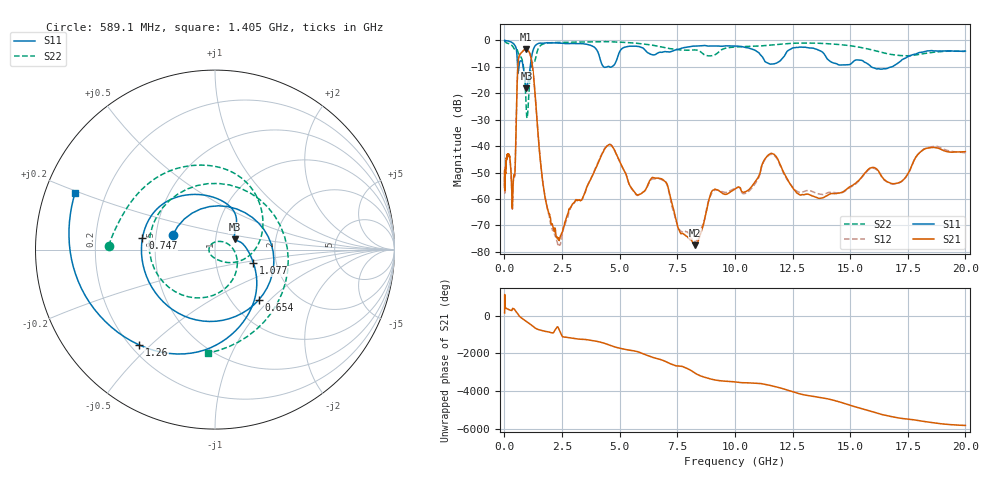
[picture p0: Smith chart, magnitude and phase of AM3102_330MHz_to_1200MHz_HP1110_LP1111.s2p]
! Date/Time: Tue, Sep 11, 2018 5:23 PM
! Network Analyzer: Agilent Technologies E8362B Rev: A.07.50.63
! Sweep from 0.010 to 20.000 GHz, 1601 Points, Sweep Type: LOG
! Power Supply: 4.949 V, 0.001 A
# Hz S DB R 50
!freq MagS11 AngS11 MagS21 AngS21 MagS12 AngS12 MagS22 AngS22
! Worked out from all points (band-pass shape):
!   1601 points, 10 MHz to 20 GHz, reference 50 ohm
!   highest |S21| = -3.32 dB at 920.7 MHz (marker M1); lowest = -77.5 dB at 8.266 GHz (marker M2)
!   |S21| within 3 dB of the highest: 627.8 MHz to 1.15 GHz (521.9 MHz wide, 58.7 % of centre)
!   lowest |S11| = -18.1 dB at 956.4 MHz (marker M3), VSWR 1.29, Z = 61.9 + j7.36 ohm
!   |S11| at or under -10 dB: 815.9 MHz to 1.118 GHz (302.1 MHz wide, 31.2 % of centre); 4.303 GHz to 4.466 GHz (163.1 MHz wide, 3.72 % of centre); 15.92 GHz to 16.81 GHz (892.5 MHz wide, 5.45 % of centre)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
!   |S22| runs from -29.5 to -0.2 dB; largest |S21 - S12| = 0.0084
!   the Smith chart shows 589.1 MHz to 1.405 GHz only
!   S11 on the Smith chart (normalised r, x): 589.1 MHz: 0.61, +0.10; 654 MHz: 1.32, -0.86; 747 MHz: 0.42, +0.07; 1.077 GHz: 1.52, -0.24; 1.26 GHz: 0.23, -0.46; 1.405 GHz: 0.09, +0.19
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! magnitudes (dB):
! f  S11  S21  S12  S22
! 10 MHz  0.0  -52.3  -52.2  -0.2
! 35.55 MHz  -0.1  -51.7  -51.9  -0.5
! 126.4 MHz  -0.2  -43.3  -44.0  -1.1
! 342.8 MHz  -1.0  -63.6  -63.8  -2.1
! 447.2 MHz  -1.8  -50.9  -51.6  -3.4
! 589.1 MHz  -12.1  -9.2  -9.2  -4.5
! 654 MHz  -8.6  -5.6  -5.8  -5.6
! 747 MHz  -7.8  -4.6  -4.6  -6.8
! 920.7 MHz  -16.8  -3.3  -3.4  -20.0
! 956.4 MHz  -18.1  -3.4  -3.5  -27.3
! 1.077 GHz  -12.9  -4.4  -4.5  -17.7
! 1.26 GHz  -3.4  -13.0  -13.0  -8.6
! 1.405 GHz  -1.5  -28.7  -29.1  -4.8
! 1.59 GHz  -1.1  -47.9  -47.9  -1.8
! 2.358 GHz  -1.0  -74.8  -77.4  -0.8
! 4.479 GHz  -9.9  -39.8  -39.6  -0.5
! 5.652 GHz  -2.2  -57.5  -57.7  -1.0
! 6.835 GHz  -4.5  -52.4  -52.7  -2.5
! 8.266 GHz  -2.2  -77.5  -76.1  -3.6
! 11.53 GHz  -9.0  -42.9  -43.2  -1.8
! 13.81 GHz  -4.5  -59.6  -58.3  -1.2
! 20 GHz  -4.0  -42.1  -42.6  -4.2
